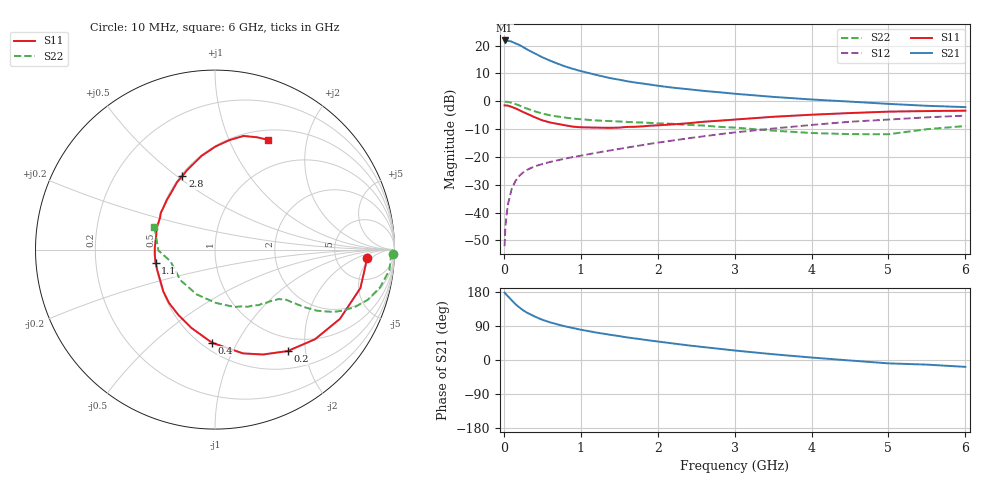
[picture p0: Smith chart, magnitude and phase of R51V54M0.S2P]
! SIEMENS Small Signal Semiconductors
! BFR183
! Si NPN RF Bipolar Junction Transistor in SOT23
! VCE = 1.5 V  IC = 4 mA
! Common Emitter S-Parameters:  May  1996
# GHz  S  MA  R  50
!  f  S11  S21  S12  S22
! GHz  MAG  ANG  MAG  ANG  MAG  ANG  MAG  ANG
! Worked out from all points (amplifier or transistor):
!   36 points, 10 MHz to 6 GHz, reference 50 ohm
!   highest |S21| = 21.9 dB at 10 MHz (marker M1)
!   |S21| within 3 dB of that: start of sweep to 288.2 MHz
!   unconditionally stable (mu >= 1): 1.108 GHz to 2.735 GHz
!   at 250 MHz: K = 0.37, MSG = 22.5 dB, |S12| = -25.6 dB
!   at 1.4 GHz: K = 1.07, MAG = 11.3 dB, |S12| = -17.6 dB
!   at 6 GHz: K = 0.91, MSG = 1.5 dB, |S12| = -5.1 dB
!   S11 on the Smith chart (normalised r, x): 10 MHz: 11, -3; 200 MHz: 0.77, -1.68; 400 MHz: 0.56, -0.80; 1.1 GHz: 0.50, -0.08; 2.8 GHz: 0.51, +0.52; 6 GHz: 0.62, +1.41
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0.01  0.8468 -3.0  12.4 178.0  0.0025 91.3  0.9914 -1.3
0.02  0.8437 -5.9  12.21 175.3  0.0056 85.3  0.9808 -2.7
0.05  0.8381 -14.8  12.26 168.7  0.0135 82.6  0.9783 -6.7
0.1  0.7959 -29.0  11.86 158.1  0.0261 75.7  0.9437 -12.9
0.15  0.7482 -41.9  10.99 147.6  0.0369 68.9  0.8959 -18.2
0.2  0.6952 -54.4  10.32 139.0  0.0456 64.3  0.8427 -22.3
0.25  0.6428 -65.4  9.445 131.3  0.0526 59.9  0.7864 -25.7
0.3  0.5989 -74.9  8.583 125.0  0.0586 57.4  0.7422 -27.9
0.4  0.5189 -91.9  7.281 114.9  0.0678 53.5  0.6632 -30.9
0.5  0.4556 -106.8  6.186 106.1  0.0748 51.8  0.6025 -32.5
0.6  0.4176 -119.2  5.384 99.5  0.0813 50.9  0.5617 -33.4
0.7  0.3925 -130.7  4.747 93.8  0.0873 51.0  0.533 -34.0
0.9  0.3507 -150.3  3.823 84.2  0.0997 52.0  0.4906 -35.0
1.1  0.3392 -167.3  3.231 76.2  0.1121 53.4  0.4648 -36.6
1.3  0.3353 178.2  2.772 69.2  0.1257 54.2  0.446 -38.2
1.6  0.3467 160.1  2.298 59.7  0.1474 54.9  0.427 -41.9
2.2  0.3857 134.0  1.757 43.6  0.1981 54.3  0.3942 -51.6
2.8  0.4486 113.9  1.456 29.6  0.2563 50.6  0.3483 -65.3
3.5  0.5274 98.2  1.202 15.2  0.3247 43.6  0.2972 -89.0
4.5  0.6155 82.5  0.988 -1.3  0.43 31.3  0.2575 -138.5
5.5  0.6681 69.5  0.831 -12.2  0.5158 18.6  0.3157 -179.1
6  0.6799 64.0  0.787 -18.1  0.5536 10.2  0.3604 159.4
